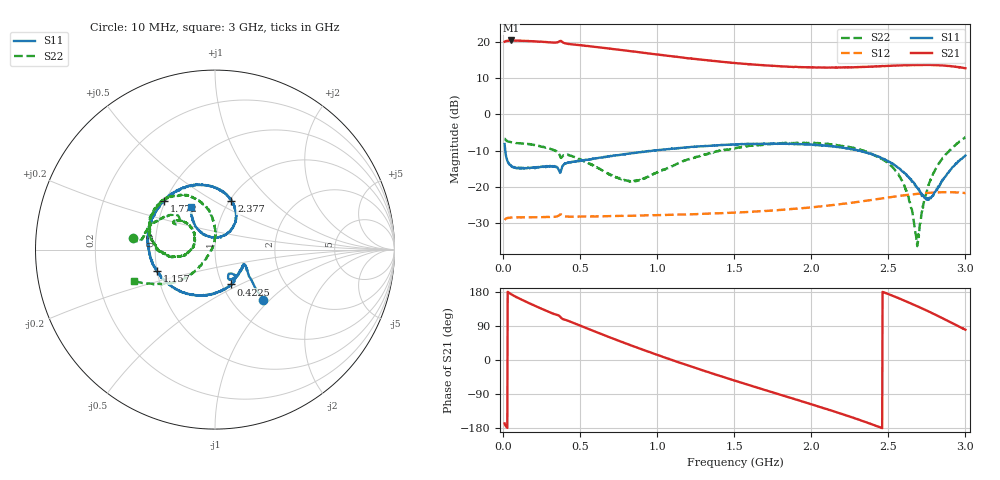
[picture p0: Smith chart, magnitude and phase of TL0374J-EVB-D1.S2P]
!Agilent Technologies,E5071C,MY46523237,B.13.01
!Date: Wed Dec 22 16:20:06 2021
!Data & Calibration Information:
!Freq	S11:SOLT2(ON)	S21:SOLT2(ON)	S12:SOLT2(ON)	S22:SOLT2(ON)
!PortZ  Port1:50+j0  Port2:50+j0
!Above PortZ is port z conversion or system Z0 setting when saving the data.
!When reading, reference impedance value at option line is always used.
# Hz S dB R 50
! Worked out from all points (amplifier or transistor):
!   1197 points, 10 MHz to 3 GHz, reference 50 ohm
!   highest |S21| = 20.5 dB at 50 MHz (marker M1)
!   |S21| within 3 dB of that: start of sweep to 832.4 MHz
!   unconditionally stable (mu >= 1): start of sweep to end of sweep
!   at 507.5 MHz: K = 1.41, MAG = 19.9 dB, |S12| = -28.3 dB
!   at 1.505 GHz: K = 1.90, MAG = 15.2 dB, |S12| = -27.1 dB
!   at 3 GHz: K = 1.30, MAG = 14.0 dB, |S12| = -21.8 dB
!   S11 on the Smith chart (normalised r, x): 10 MHz: 1.38, -0.92; 422.5 MHz: 1.10, -0.45; 1.157 GHz: 0.50, -0.14; 1.772 GHz: 0.49, +0.32; 2.377 GHz: 1.02, +0.60; 3 GHz: 0.69, +0.35
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1e7  -8.17 -46.4  20.12 -167.3  -29.20 26.8  -6.74 172.1
5e7  -14.15 -28.9  20.47 174.2  -28.53 2.1  -7.67 172.5
1.475e8  -14.87 -31.1  20.34 154.5  -28.46 -9.6  -8.17 162.8
2.45e8  -14.50 -45.8  20.13 136.1  -28.42 -18.3  -8.85 153.6
3.75e8  -15.75 -54.9  20.36 112.0  -27.68 -30.2  -12.03 142.5
4.225e8  -13.38 -65.1  19.52 103.4  -28.28 -35.0  -11.23 144.3
5.1e8  -12.63 -80.0  19.14 89.1  -28.24 -41.7  -12.58 138.4
6.4e8  -11.91 -97.7  18.49 68.0  -28.18 -52.6  -15.38 138.2
7.6e8  -11.14 -113.6  17.87 49.4  -28.06 -62.5  -17.74 150.6
8.725e8  -10.51 -126.9  17.26 32.4  -27.98 -72.3  -18.39 173.4
1.0075e9  -9.85 -142.5  16.56 12.5  -27.84 -83.5  -15.89 -171.8
1.1575e9  -9.23 -159.6  15.81 -8.5  -27.67 -96.2  -13.23 -169.6
1.335e9  -8.68 -178.7  14.93 -32.6  -27.43 -111.2  -10.74 -175.9
1.505e9  -8.36 163.4  14.22 -54.7  -27.13 -125.8  -9.33 174.1
1.7725e9  -8.12 135.9  13.41 -88.4  -26.52 -148.9  -8.10 157.0
2.005e9  -8.33 111.7  13.04 -117.5  -25.67 -170.0  -7.98 139.8
2.3775e9  -10.85 71.5  13.21 -167.5  -23.74 151.6  -10.66 109.7
2.5025e9  -13.07 57.4  13.45 173.5  -22.95 136.0  -13.70 97.3
2.6875e9  -20.32 57.6  13.67 141.9  -21.97 109.1  -36.44 140.3
2.7975e9  -21.72 114.1  13.66 121.1  -21.58 90.9  -15.94 -132.9
2.9e9  -15.49 129.9  13.38 100.2  -21.51 73.2  -9.93 -144.7
3e9  -11.36 119.0  12.79 79.9  -21.75 55.2  -6.30 -158.7
